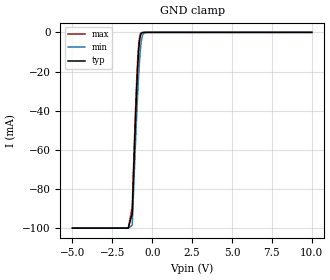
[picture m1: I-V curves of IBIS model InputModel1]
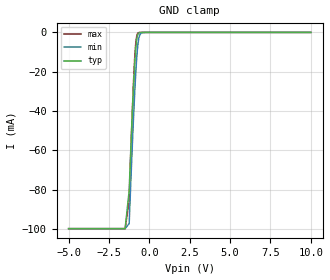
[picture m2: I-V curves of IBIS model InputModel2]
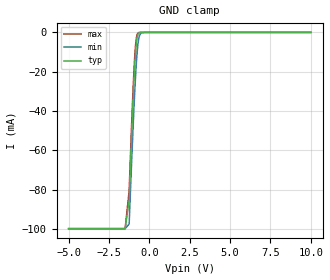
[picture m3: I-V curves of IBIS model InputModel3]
[IBIS Ver]   2.1
[File name]   e_001bx5.ibs   | e_= TSOP, 001bx= abbr chip name, 5= 5V Vcc
[File Rev]   2.00
[Date]   7-February-1996
[Source]   File generated from simulation at Intel Corporation
[Notes]   This IBIS model is for the 28F001BX-T and 28F001BX-B.
   Rev 2.00 uses actual measurements found in a lab.
[Disclaimer] INTEL DEVELOPER'S SOFTWARE LICENSE AGREEMENT
| BY USING THIS SOFTWARE, YOU ARE AGREEING TO BE BOUND
| BY THE TERMS OFTHIS AGREEMENT.  DO NOT USE THE SOFTWARE
| UNTIL YOU HAVE CAREFULLY READAND AGREED TO THE FOLLOWING
| TERMS AND CONDITIONS.  IF YOU DO NOT AGREETO THE TERMS
| OF THIS AGREEMENT, PROMPTLY RETURN THE SOFTWARE PACKAGE
| ANDANY ACCOMPANYING ITEMS.
| IF YOU USE THIS SOFTWARE, YOU WILL BE BOUND BY THE TERMS
| OF THIS AGREEMENT
| LICENSE: Intel Corporation ("Intel") grants you the non-exclusive right
| to use the enclosed software program ("Software").  You will not use,
| copy, modify, rent, sell or transfer the Software or any portion
| thereof, except as provided in this Agreement.
| System OEM Developers may:
| 1.   Copy the Software for support, backup or archival purposes;
| 2.   Install, use, or distribute Intel owned Software in object code
|   only;
| 3.   Modify and/or use Software source code that Intel directly makes
|   available to you as an OEM Developer;
| 4.   Install, use, modify, distribute, and/or make or have made
|   derivatives ("Derivatives") of Intel owned Software under the
|   terms and conditions in this Agreement, ONLY if you are a System
|   OEM Developer and NOT an end-user.
| RESTRICTIONS:
| YOU WILL NOT:
| 1.   Copy the Software, in whole or in part, except as provided for
|   in this Agreement;
| 2.   Decompile or reverse engineer any Software provided in object
|   code format;
| 3.   Distribute any Software or Derivative code to any end-users,
|   unless approved by Intel in a prior writing.
| TRANSFER: You may transfer the Software to another OEM
| Developer if thereceiving party agrees to the terms of this
| Agreement at the sole risk of any receiving party.
| OWNERSHIP AND COPYRIGHT OF SOFTWARE:
| Title to the Software and all copies thereof remain with Intel
| or its vendors.  The Software iscopyrighted and is protected by
| United States and international copyright laws.  You will not
| remove the copyright notice from the Software.  You agree to
| prevent any unauthorized copying of the Software.
| DERIVATIVE WORK: OEM Developers that make or have made
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[Copyright]   Copyright 1996, Intel Corporation, All Rights Reserved|
[Component]   E28F001BX   | 32-lead TSOP package, 28F001BX
[Manufacturer]  Intel   | Boot Block(tm) Memory
|   | operating in 5V Vcc range
[Package]
| The following values apply for the Alloy-42 leadframe.
|Variable   typ   min   max
R_pkg   122.5m   112m   133m
L_pkg   7.35nH   6.86nH   7.84nH
C_pkg   0.87pF   0.80pF   0.94pF
|***************************Pin Defintions***********************************
[Pin]   signal_name   model_name   R_pin   L_pin   C_pin
  1   A11   InputModel5
  2   A09   InputModel3
  3   A08   InputModel2
  4   A13   InputModel1
  5   A14   InputModel1
  6   RP#   InputModel7
  8   VCC   POWER
  9   VPP   POWER
 10   A16   InputModel1
 11   A15   InputModel1
 12   A12   InputModel1
 13   A07   InputModel1
 14   A06   InputModel1
 15   A05   InputModel1
 16   A04   InputModel1
 17   A03   InputModel1
 18   A02   InputModel1
 19   A01   InputModel1
 20   A00   InputModel1
 21   DQ0   InputOutput
 22   DQ1   InputOutput
 23   DQ2   InputOutput
 24   GND   GND
 25   DQ3   InputOutput
 26   DQ4   InputOutput
 27   DQ5   InputOutput
 28   DQ6   InputOutput
 29   DQ7   InputOutput
 30   CE#   InputModel6
 31   WE#   InputModel6
 32   VCC   Power
| Models and submodels in the file (8): InputModel1 (Input), InputModel2 (Input), InputModel3 (Input), InputModel4 (Input), InputModel5 (Input), InputModel6 (Input), InputModel7 (Input), InputOutput (I/O)
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|**********************Input Model 1****************************************
[Model]   InputModel1
Model_type   Input
|   Model for pins A[0:7] and A[12:16]
Vinl = 0.8V
Vinh = 2.0V
|Variable   Typ   Min   Max
C_comp   9.13p   7.20p   11.06p
[Voltage Range]   5.0V   4.5V   5.5V
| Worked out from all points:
|   GND clamp passes 1 mA (typ) near -0.71 V on its own axis
[GND_clamp]
|Voltage   I(typ)   I(min)   I(max)
-5V       -99.85mA   -99.85mA   -99.85mA
-1.5V     -99.85mA   -99.85mA   -99.85mA
-1.25V    -92.41mA   -98.35mA   -88.66mA
-1.1V     -56.22mA   -67.11mA   -51.63mA
-950mV    -24.52mA   -38.21mA   -20.03mA
-900mV    -16.1mA    -29.62mA   -12.04mA
-850mV    -9.506mA   -21.94mA   -6.298mA
-800mV    -4.773mA   -15.11mA   -2.664mA
-700mV    -757.1uA   -5.52mA    -292.9uA
-600mV    -77.96uA   -1.375mA   -29.35uA
-250mV    0A         0A         0A
10V       0A         0A         0A
[Power_clamp]
| Input buffer circuits of this product do not intrinisically
| require a [Power_clamp] defintion.  This zero current
| [Power_clamp] table is provided for compatibility with
| some IBIS parsers.
|Voltage   I(typ)   I(min)   I(max)
-5V       0A         0A         0A
0V        0A         0A         0A
5V        0A         0A         0A
10V       0A         0A         0A
|**********************Input Model 2**********************************
[Model]   InputModel2
Model_type   Input
|   Model for pin A[8]
Vinl = 0.8V
Vinh = 2.0V
|Variable   Typ   Min   Max
C_comp   9.13p   7.20p   11.06p
[Voltage Range]   5.0V   4.5V   5.5V
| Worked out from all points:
|   GND clamp passes 1 mA (typ) near -0.71 V on its own axis
[GND_clamp]
|Voltage   I(typ)   I(min)   I(max)
-5V       -99.85mA   -99.85mA   -99.85mA
-1.5V     -99.85mA   -99.85mA   -99.85mA
-1.25V    -80.64mA   -97.24mA   -85.74mA
-1.05V    -39.78mA   -56.59mA   -39.22mA
-950mV    -22.19mA   -37.94mA   -19.68mA
-900mV    -14.83mA   -29.45mA   -11.9mA
-850mV    -8.947mA   -21.86mA   -6.262mA
-800mV    -4.637mA   -15.1mA    -2.671mA
-700mV    -770.9uA   -5.542mA   -297.9uA
-600mV    -82.05uA   -1.388mA   -30.72uA
-250mV    0A         0A         0A
10V       0A         0A         0A
[Power_clamp]
| Input buffer circuits of this product do not intrinisically
| require a [Power_clamp] defintion.  This zero current
| [Power_clamp] table is provided for compatibility with
| some IBIS parsers.
|Voltage   I(typ)   I(min)   I(max)
-5V       0A         0A         0A
0V        0A         0A         0A
5V        0A         0A         0A
10V       0A         0A         0A
|*********************Input Model 3*********************************
[Model]   InputModel3
Model_type   Input
|   Model for pin A[9]
Vinl = 0.8V
Vinh = 2.0V
|Variable   Typ   Min   Max
C_comp   9.13p   7.20p   11.06p
[Voltage Range]   5.0V   4.5V   5.5V
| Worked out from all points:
|   GND clamp passes 1 mA (typ) near -0.71 V on its own axis
[GND_clamp]
|Voltage   I(typ)   I(min)   I(max)
-5V       -99.85mA   -99.85mA   -99.85mA
-1.5V     -99.85mA   -99.85mA   -99.85mA
-1.25V    -85.38mA   -97.47mA   -80.58mA
-1.05V    -42.22mA   -56.76mA   -37.24mA
-950mV    -23.59mA   -38.06mA   -18.92mA
-900mV    -15.77mA   -29.54mA   -11.58mA
-850mV    -9.508mA   -21.93mA   -6.173mA
-800mV    -4.907mA   -15.14mA   -2.678mA
-700mV    -819.1uA   -5.554mA   -304.4uA
-600mV    -87.72uA   -1.392mA   -31.35uA
-250mV    0A         0A         0A
10V       0A         0A         0A
[Power_clamp]
| Input buffer circuits of this product do not intrinisically
| require a [Power_clamp] defintion.  This zero current
| [Power_clamp] table is provided for compatibility with
| some IBIS parsers.
|Voltage   I(typ)   I(min)   I(max)
-5V       0A         0A         0A
0V        0A         0A         0A
5V        0A         0A         0A
10V       0A         0A         0A
